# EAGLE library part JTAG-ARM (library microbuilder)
20 Pin JTAG Connector For use with ARM7, and ARM9. Supported by some Cortex M3 boards with SWJ-DP interfaces (dual SWP/JTAG support). 4UConnector: 03556
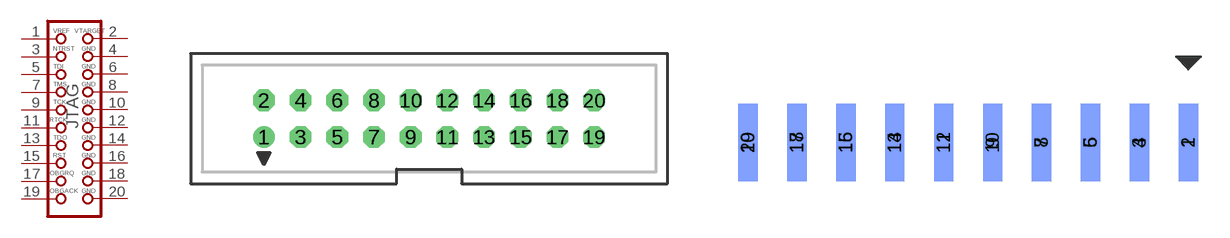
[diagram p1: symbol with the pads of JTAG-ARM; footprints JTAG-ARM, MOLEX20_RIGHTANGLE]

Designator prefix JTAG

## JTAG-ARM  [JTAG-ARM]
1  1  pas
2  2  pas
3  3  pas
4  4  pas
5  5  pas
6  6  pas
7  7  pas
8  8  pas
9  9  pas
10  10  pas
11  11  pas
12  12  pas
13  13  pas
14  14  pas
15  15  pas
16  16  pas
17  17  pas
18  18  pas
19  19  pas
20  20  pas

## JTAG-ARMEDGE  [MOLEX20_RIGHTANGLE]
Pads as for JTAG-ARM

## Footprint JTAG-ARM (pad centres in mm)
20 Pin JTAG Connector (ARM7, ARM9)
drill 1: 1 -11.43,-1.27
drill 1 octagon: 2 -11.43,1.27; 3 -8.89,-1.27; 4 -8.89,1.27; 5 -6.35,-1.27; 6 -6.35,1.27; 7 -3.81,-1.27; 8 -3.81,1.27; 9 -1.27,-1.27; 10 -1.27,1.27; 11 1.27,-1.27; 12 1.27,1.27; 13 3.81,-1.27; 14 3.81,1.27; 15 6.35,-1.27; 16 6.35,1.27; 17 8.89,-1.27; 18 8.89,1.27; 19 11.43,-1.27; 20 11.43,1.27

## Footprint MOLEX20_RIGHTANGLE (pad centres in mm)
Molex 20 Pin Header Footprint designed to mount connector on edge of board, one row on top layer, one row on bottom layer
smd 1 x 4: 1 11.43,0; 3 8.89,0; 5 6.35,0; 7 3.81,0; 9 1.27,0; 11 -1.27,0; 13 -3.81,0; 15 -6.35,0; 17 -8.89,0; 19 -11.43,0
smd 1 x 4 bottom: 2 11.43,0; 4 8.89,0; 6 6.35,0; 8 3.81,0; 10 1.27,0; 12 -1.27,0; 14 -3.81,0; 16 -6.35,0; 18 -8.89,0; 20 -11.43,0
